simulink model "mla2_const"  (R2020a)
settings: Solver=ode5  StartTime=0.0  StopTime=2  FixedStep=0.0001  RelTol=1e-4  EnableMultiTasking=on
PreLoadFcn:
  | MLA_Sensor1 = load('mla_sensor1.dat');
libraries: libmla x1

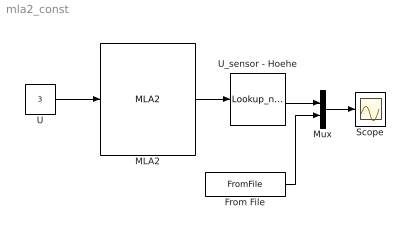
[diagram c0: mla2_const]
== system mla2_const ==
  From File : FromFile  FileName=mla_const.mat  SampleTime=0
  MLA2 : libmla/MLA2  g=9.81  m=0.125  Fr_g=0.14  Fr_h=0.1  d_l=0.14  d_t=0.09  a=40691  b=0.0687  N=4.282
  Mux : Mux  Inputs=2
  Scope : Scope
  U : Constant  Value=3
  U_sensor - Hoehe : Lookup_n-D  NumberOfTableDimensions=1  BreakpointsForDimension1=MLA_Sensor1(:,1)  Table=MLA_Sensor1(:,2)  RndMeth=Simplest
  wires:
  MLA2/1 -> U_sensor - Hoehe/1
  U/1 -> MLA2/1
  U_sensor - Hoehe/1 -> Mux/1
  Mux/1 -> Scope/1
  From File/1 -> Mux/2
